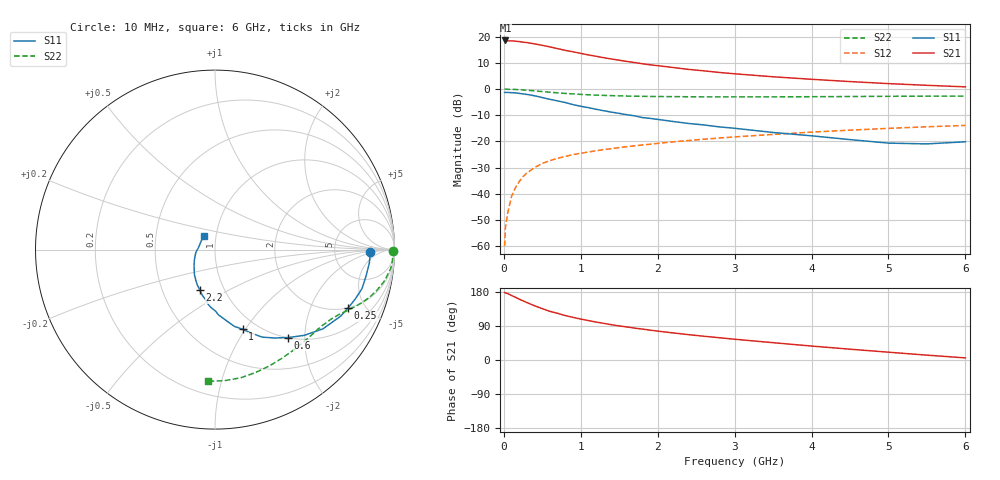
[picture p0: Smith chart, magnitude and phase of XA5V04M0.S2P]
! SIEMENS Discrete & RF Semiconductors
! BFY180
! Si NPN RF Bipolar Junction Transistor in MICRO-X
! VCE = 5 V  IC = 4 mA
! Common Emitter S-Parameters:  May  1997
# GHz  S  MA  R  50
!  f  S11  S21  S12  S22
! GHz  MAG  ANG  MAG  ANG  MAG  ANG  MAG  ANG
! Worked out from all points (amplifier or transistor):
!   36 points, 10 MHz to 6 GHz, reference 50 ohm
!   highest |S21| = 18.6 dB at 20 MHz (marker M1)
!   |S21| within 3 dB of that: start of sweep to 680.7 MHz
!   unconditionally stable (mu >= 1): 2.06 GHz to end of sweep
!   at 250 MHz: K = 0.20, MSG = 25.7 dB, |S12| = -33.4 dB
!   at 1.4 GHz: K = 0.86, MSG = 17.1 dB, |S12| = -22.7 dB
!   at 6 GHz: K = 1.06, MAG = 5.8 dB, |S12| = -13.9 dB
!   S11 on the Smith chart (normalised r, x): 10 MHz: 13, -1; 250 MHz: 1.98, -3.75; 600 MHz: 1.01, -1.66; 1 GHz: 0.85, -0.97; 2.2 GHz: 0.77, -0.37; 6 GHz: 0.87, +0.13
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0.01  0.8619 -0.9  8.427 178.2  0.001 85.8  0.9923 -0.3
0.02  0.8648 -1.9  8.494 177.3  0.0022 88.3  0.9999 -0.8
0.05  0.8632 -4.9  8.342 175.1  0.0043 84.7  0.992 -2.1
0.1  0.8547 -9.7  8.345 170.3  0.0089 85.3  0.9891 -4.2
0.2  0.829 -19.3  8.087 160.6  0.0171 79.0  0.9729 -8.1
0.25  0.8092 -23.8  7.886 156.1  0.0213 76.8  0.9635 -10.0
0.3  0.7918 -28.0  7.736 151.5  0.025 73.7  0.95 -11.7
0.4  0.7459 -36.3  7.301 143.1  0.0317 69.8  0.9254 -14.7
0.5  0.6894 -43.9  6.856 135.4  0.0381 66.1  0.8968 -17.5
0.6  0.6376 -50.2  6.388 128.3  0.0431 63.7  0.8711 -19.8
0.8  0.5537 -61.7  5.489 117.2  0.0518 59.2  0.8265 -23.4
1  0.4698 -70.8  4.815 108.0  0.0595 56.0  0.7926 -26.5
1.1  0.442 -75.7  4.493 104.0  0.0629 55.2  0.7792 -27.7
1.3  0.3856 -83.2  3.97 96.7  0.0701 53.2  0.7581 -30.3
1.5  0.3438 -89.3  3.56 89.9  0.0763 51.9  0.7429 -32.9
1.7  0.3084 -97.0  3.216 84.1  0.0825 50.8  0.7315 -35.4
2.2  0.2408 -110.6  2.587 71.5  0.0983 47.9  0.7179 -41.9
2.8  0.1899 -125.8  2.081 58.8  0.1162 44.5  0.7112 -49.5
3.5  0.1484 -141.8  1.72 45.7  0.1363 39.8  0.7113 -58.5
4.5  0.1085 -170.9  1.392 28.5  0.1644 32.6  0.7213 -71.8
5.5  0.0898 153.3  1.181 12.8  0.1907 24.9  0.7323 -86.0
6  0.0986 130.5  1.103 5.5  0.2027 20.7  0.7344 -93.1
